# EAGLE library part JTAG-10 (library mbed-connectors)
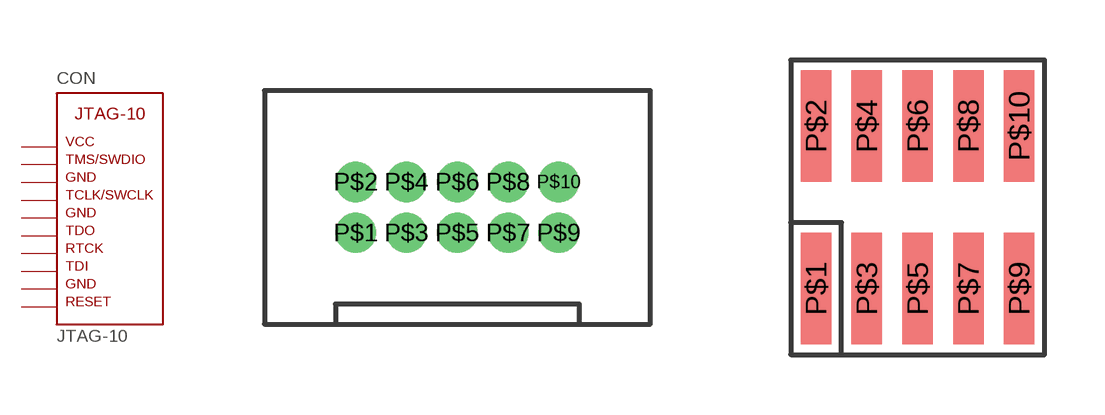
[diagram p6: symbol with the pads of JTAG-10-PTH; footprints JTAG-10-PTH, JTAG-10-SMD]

Designator prefix CON

## JTAG-10_PTH  [JTAG-10-PTH]
P$1  P$1
P$2  P$2
P$3  P$3
P$4  P$4
P$5  P$5
P$6  P$6
P$7  P$7
P$8  P$8
P$9  P$9
P$10  P$10

## JTAG-10_SMD  [JTAG-10-SMD]
Pads as for JTAG-10-PTH

## Footprint JTAG-10-PTH (pad centres in mm)
drill 0.5 pad 0.813: P$1 0,0; P$2 0,1.27; P$3 1.27,0; P$4 1.27,1.27; P$5 2.54,0; P$6 2.54,1.27; P$7 3.81,0; P$8 3.81,1.27; P$9 5.08,0; P$10 5.08,1.27

## Footprint JTAG-10-SMD (pad centres in mm)
smd 0.762 x 2.794: P$1 0.381,-2.032; P$2 0.381,2.032; P$3 1.651,-2.032; P$4 1.651,2.032; P$5 2.921,-2.032; P$6 2.921,2.032; P$7 4.191,-2.032; P$8 4.191,2.032; P$9 5.461,-2.032; P$10 5.461,2.032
